FUNCTION FC 1021 : VOID
TITLE =Step Reset
//Resets alle bits sequential to the adres given by P##first_bit
//This pointer has to be in a DB (eg of type array [1..32] of bool)
//max_bits gives the amount of bits to be resettet
AUTHOR : PCR
FAMILY : Step
VERSION : 1.0


VAR_INPUT
  first_bit : POINTER ;
  max_bits : INT ;
END_VAR
VAR_TEMP
  count : INT ;
  workblock : INT ;
  command_pointer : DWORD ;
END_VAR
BEGIN
NETWORK
TITLE =Open DB
//return if pointer is not in a DB!
      SET   ;
      SAVE  ;
      L     P##first_bit;
      LAR1  ;
      L     W [AR1,P#0.0];
      T     #workblock;
      L     0;
      ==I   ;
      BEC   ;
      OPN   DB [#workblock];
NETWORK
TITLE =reset step

      L     D [AR1,P#2.0]; //Type,byte,bit
      AD    DW#16#7FFF8; //Delete type and bit
      T     #command_pointer; //Save pointer byte
      LAR1  ; //AR1 is pointer to byte 1

      L     #max_bits; //set counter
loop: T     #count;
      R     DBX [AR1,P#0.0]; //reset bit            //check or step, step[#count], is high
      +AR1  P#0.1; //increase pointer
      LOOP  loop; //count -1, if not 0 jump loop

      SET   ;
      SAVE  ;
END_FUNCTION

FUNCTION FC 1022 : VOID
TITLE =Step calculation
//Finds the first bit after the adres given by P##first_bit that is TRUE.
//This pointer has to be in a DB (eg of type array [1..32] of bool)
//max_bits gives the amount of bits to be searched.
//bit_number gives the number of the first bit that is TRUE.
AUTHOR : PCR
FAMILY : Step
VERSION : 1.0


VAR_INPUT
  first_bit : POINTER ;
  max_bits : INT ;
END_VAR
VAR_OUTPUT
  bit_number : INT ;
END_VAR
VAR_TEMP
  count : INT ;
  workblock : INT ;
  command_pointer : DWORD ;
END_VAR
BEGIN
NETWORK
TITLE =Open DB
//return if pointer is not in a DB!
      SET   ;
      SAVE  ;
      L     P##first_bit;
      LAR1  ;
      L     W [AR1,P#0.0];
      T     #workblock;
      L     0;
      ==I   ;
      BEC   ;
      OPN   DB [#workblock];
NETWORK
TITLE =Check step

      L     D [AR1,P#2.0]; //Type,byte,bit
      AD    DW#16#7FFF8; //Delete type and bit
      T     #command_pointer; //Save pointer byte
      LAR1  ; //AR1 is pointer to byte 1

      L     #max_bits; //set counter
loop: T     #count;
      A     DBX [AR1,P#0.0]; //check or step, step[#count], is high
      JC    disp; //if high then jump to write to output
      +AR1  P#0.1; //increase pointer
      LOOP  loop; //count -1, if not 0 jump loop

      T     #bit_number; //no bit found = 0
      BE    ;

disp: L     #max_bits; //last
      L     #count; //minus counter
      -I    ;
      INC   1; //add 1 (remove wenn starting with '0'
//      L     1// use this wenn #max_bits can be greater then 255 (INC is bytecount)
//      +I     //
      T     #bit_number; // write step number to output

      SET   ;
      SAVE  ;
END_FUNCTION

FUNCTION FC 1023 : VOID
TITLE =step function
//EN input: step condition
//Step_EN : enable to step, wil be resetet after step
//Step_act: Actual step active, wil be resetet after step
//Step_new: Step to go to, wil be set after step
//ENO out : Step actions (One Shot!)
AUTHOR : PCR
FAMILY : Step
VERSION : 1.0


VAR_IN_OUT
  Step_EN : BOOL ;
  Step_act : BOOL ;
  Step_new : BOOL ;
END_VAR
VAR_TEMP
  ENO : BOOL ;
END_VAR
BEGIN
NETWORK
TITLE =next step

      A     #Step_EN;
      A     #Step_act;
      =     #ENO;
      R     #Step_EN;
      R     #Step_act;
      S     #Step_new;
NETWORK
TITLE =Set ENO

      A     #ENO;
      SAVE  ;
END_FUNCTION

FUNCTION FC 1024 : VOID
TITLE =step function
//EN input  : step condition
//Choice    : Condition for the new step
//Step_EN   : enable to step, wil be resetet after step
//Step_act  : Actual step active, wil be resetet after step
//Step_new_1: Step to go to wenn Choice is true, wil be set after step
//Step_new_0: Step to go to wenn Choice is false, wil be set after step
//ENO out   : Step actions (One Shot!)
AUTHOR : PCR
FAMILY : Step
VERSION : 1.0


VAR_INPUT
  Choice : BOOL ;
END_VAR
VAR_IN_OUT
  Step_EN : BOOL ;
  Step_act : BOOL ;
  Step_new_1 : BOOL ;
  Step_new_0 : BOOL ;
END_VAR
VAR_TEMP
  ENO : BOOL ;
END_VAR
BEGIN
NETWORK
TITLE =next step
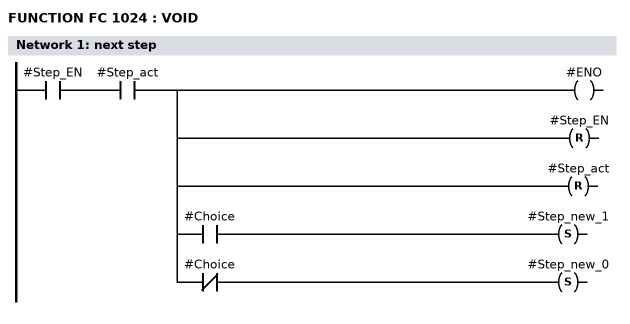
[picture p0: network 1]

      A     #Step_EN;
      A     #Step_act;
      =     L      1.0;
      A     L      1.0;
      BLD   102;
      =     #ENO;
      A     L      1.0;
      BLD   102;
      R     #Step_EN;
      A     L      1.0;
      BLD   102;
      R     #Step_act;
      A     L      1.0;
      A     #Choice;
      S     #Step_new_1;
      A     L      1.0;
      AN    #Choice;
      S     #Step_new_0;
NETWORK
TITLE =Set ENO

      A     #ENO;
      SAVE  ;
END_FUNCTION

FUNCTION FC 1025 : VOID
TITLE =Step Reset/Calculate
//Finds the LAST bit after the adres given by P##first_bit that is TRUE.
//If 'reset' is high all bits sequential to the adres given by P##first_bit
//
//The pointer has to be in a DB (eg of type array [1..xx] of bool)
//max_bits gives the amount of bits to be searched or resettet.
//bit_number gives the number of the bit that is TRUE.
AUTHOR : PCR
FAMILY : Step
VERSION : 1.0


VAR_INPUT
  first_bit : POINTER ;
  max_bits : INT ;
  reset : BOOL ;
END_VAR
VAR_OUTPUT
  bit_number : INT ;
END_VAR
VAR_TEMP
  count : INT ;
  workblock : INT ;
  command_pointer : DWORD ;
END_VAR
BEGIN
NETWORK
TITLE =Open DB
//return if pointer is not in a DB!
      SET   ;
      SAVE  ;
      L     P##first_bit;
      LAR1  ;
      L     W [AR1,P#0.0];
      T     #workblock;
      L     0;
      T     #bit_number; // write '0' to output, has nothing to do with the DB!
      ==I   ;
      BEC   ;
      OPN   DB [#workblock];
NETWORK
TITLE =reset and calculate step

      L     D [AR1,P#2.0]; //Type,byte,bit
      AD    DW#16#7FFF8; //Delete type and bit
      T     #command_pointer; //Save pointer byte
      LAR1  ; //AR1 is pointer to byte 1

      L     #max_bits; //set counter
loop: T     #count;
      A     #reset;
      R     DBX [AR1,P#0.0]; //reset bit if #reset is high
      A     DBX [AR1,P#0.0]; //check or step, step[#count], is high
      JCN   Nwrt; //if not high then jump over write to output
      L     #max_bits; //last
      L     #count; //minus counter
      -I    ;
      +     1; //add 1 (remove wenn starting with '0')
      T     #bit_number; //write step number to output

      L     #count; //#count has to be loaded
Nwrt: +AR1  P#0.1; //increase pointer with 1 bit
      LOOP  loop; //count -1, if not 0 jump loop
NETWORK
TITLE =Reset to ENO (for more resets or sets)

      A     #reset;
      SAVE  ;
END_FUNCTION

FUNCTION_BLOCK FB 1
TITLE =Step program
VERSION : 0.1


VAR_INPUT
  Start : BOOL ;
  Reset : BOOL ;
END_VAR
VAR
  step : ARRAY  [1 .. 32 ] OF BOOL ;
  step_nr : INT ;
  Step_active : BOOL ;
END_VAR
VAR_TEMP
  step_EN : BOOL ;
  Condition1 : BOOL ;
  Condition2 : BOOL ;
  Condition3 : BOOL ;
  condition4 : BOOL ;
  condition5 : BOOL ;
  Action1 : BOOL ;
  Action2 : BOOL ;
  Action3 : BOOL ;
END_VAR
BEGIN
NETWORK
TITLE =Calculate active step and Reset all step and actions if needed.
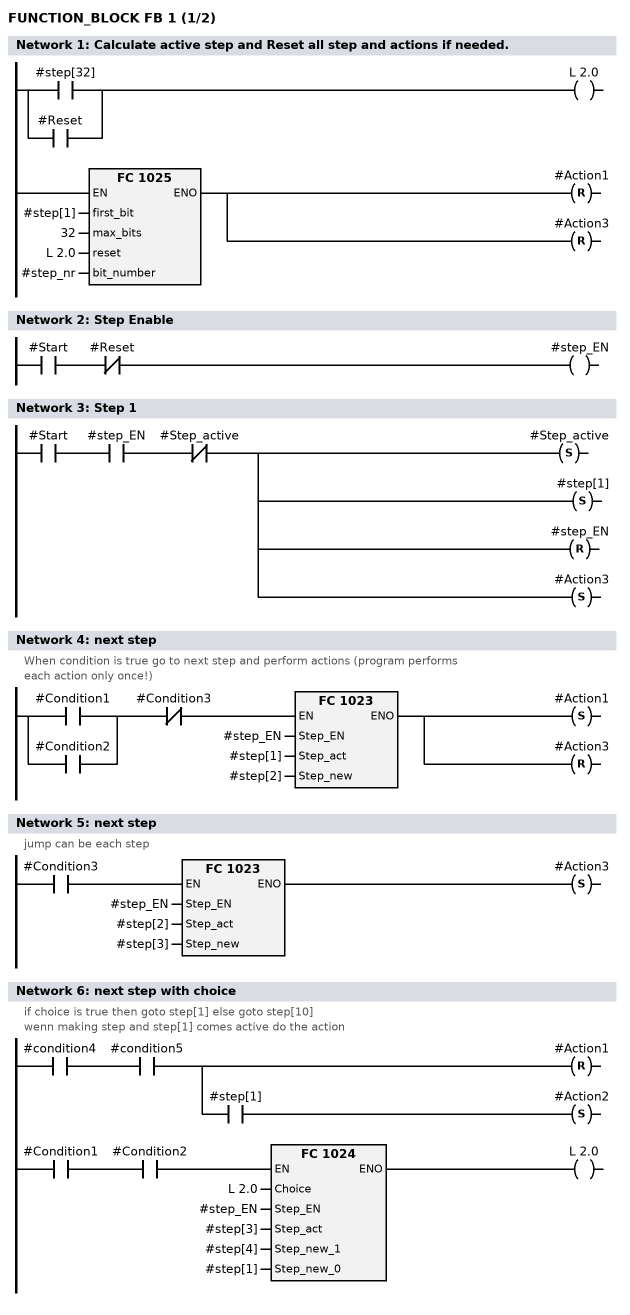
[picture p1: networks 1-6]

      A(    ;
      O     #step[32];
      O     #Reset;
      )     ;
      =     L      2.0;
      BLD   103;
      CALL FC  1025 (
           first_bit                := #step[1],
           max_bits                 := 32,
           reset                    := L      2.0,
           bit_number               := #step_nr);
      A     BR;
      R     #Action1;
      R     #Action3;
NETWORK
TITLE =Step Enable

      A     #Start;
      AN    #Reset;
      =     #step_EN;
NETWORK
TITLE =Step 1

      A     #Start;
      A     #step_EN;
      AN    #Step_active;
      S     #Step_active;
      S     #step[1];
      R     #step_EN;
      S     #Action3;
NETWORK
TITLE =next step
//When condition is true go to next step and perform actions (program performs
//each action only once!)
      A(    ;
      O     #Condition1;
      O     #Condition2;
      )     ;
      AN    #Condition3;
      JNB   _001;
      CALL FC  1023 (
           Step_EN                  := #step_EN,
           Step_act                 := #step[1],
           Step_new                 := #step[2]);
_001: A     BR;
      S     #Action1;
      R     #Action3;
NETWORK
TITLE =next step
//jump can be each step
      A     #Condition3;
      JNB   _002;
      CALL FC  1023 (
           Step_EN                  := #step_EN,
           Step_act                 := #step[2],
           Step_new                 := #step[3]);
_002: A     BR;
      S     #Action3;
NETWORK
TITLE =next step with choice
//if choice is true then goto step[1] else goto step[10]
//wenn making step and step[1] comes active do the action
      A     #condition4;
      A     #condition5;
      =     L      2.0;
      BLD   103;
      A     #Condition1;
      A     #Condition2;
      JNB   _003;
      CALL FC  1024 (
           Choice                   := L      2.0,
           Step_EN                  := #step_EN,
           Step_act                 := #step[3],
           Step_new_1               := #step[4],
           Step_new_0               := #step[1]);
_003: A     BR;
      =     L      2.0;
      A     L      2.0;
      BLD   102;
      R     #Action1;
      A     L      2.0;
      A     #step[1];
      S     #Action2;
NETWORK
TITLE =last step (jump)
//jump can be each step
//step[32] is used to reset the program
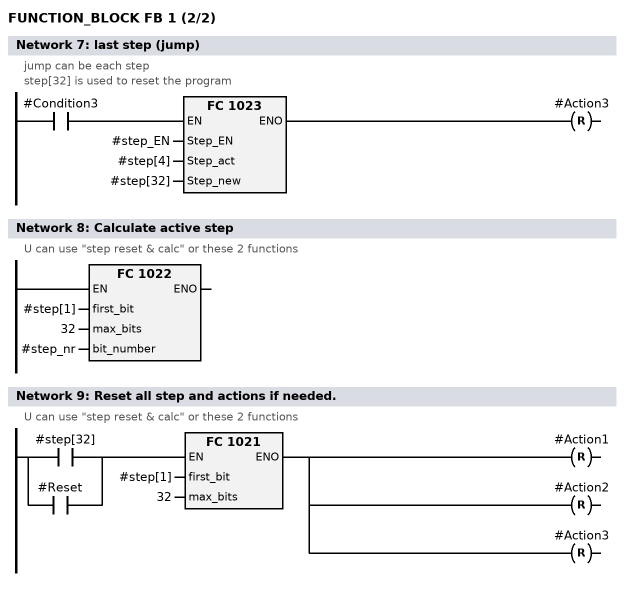
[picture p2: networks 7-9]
      A     #Condition3;
      JNB   _004;
      CALL FC  1023 (
           Step_EN                  := #step_EN,
           Step_act                 := #step[4],
           Step_new                 := #step[32]);
_004: A     BR;
      R     #Action3;
NETWORK
TITLE =Calculate active step
//U can use "step reset & calc" or these 2 functions
      CALL FC  1022 (
           first_bit                := #step[1],
           max_bits                 := 32,
           bit_number               := #step_nr);
      NOP   0;
NETWORK
TITLE =Reset all step and actions if needed.
//U can use "step reset & calc" or these 2 functions
      A(    ;
      O     #step[32];
      O     #Reset;
      )     ;
      JNB   _005;
      CALL FC  1021 (
           first_bit                := #step[1],
           max_bits                 := 32);
_005: A     BR;
      R     #Action1;
      R     #Action2;
      R     #Action3;
END_FUNCTION_BLOCK

